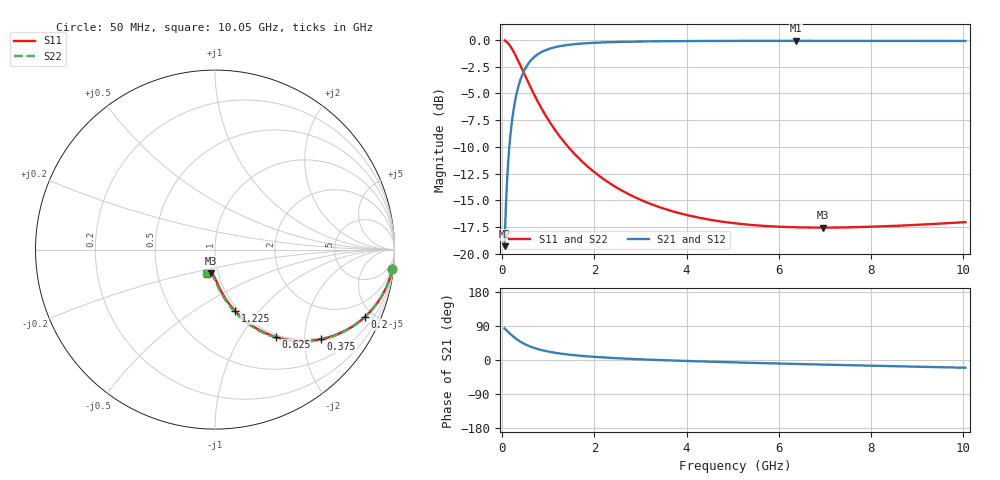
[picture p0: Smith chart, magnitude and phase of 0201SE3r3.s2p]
! AVX Thin Film Operation		Date: August 2001
! Description: Accu-P® Series, Thin Film, SMD, RF Capacitor
! Part Number: 0201YJ3R3ABW
! 50 MHz  -  10.05 GHz
! Serial Measurements
# mhz S db R 50
!	S11		S21		S12		S22
!	dB	Phase	dB	Phase	dB	Phase	dB	Phase
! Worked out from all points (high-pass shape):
!   401 points, 50 MHz to 10.05 GHz, reference 50 ohm
!   highest |S21| = -0.09 dB at 6.375 GHz (marker M1); lowest = -19.3 dB at 50 MHz (marker M2)
!   |S21| within 3 dB of the highest: 451.6 MHz to end of sweep
!   lowest |S11| = -17.5 dB at 6.95 GHz (marker M3), VSWR 1.31, Z = 46.1 - j12.2 ohm
!   |S11| at or under -10 dB: 1.431 GHz to end of sweep
!   |S22| runs from -17.5 to -0.1 dB; largest |S21 - S12| = 0
!   S11 on the Smith chart (normalised r, x): 50 MHz: 1, -18; 200 MHz: 0.96, -4.48; 375 MHz: 0.96, -2.40; 625 MHz: 0.96, -1.44; 1.225 GHz: 0.96, -0.75; 10.05 GHz: 0.88, -0.24
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50  -0.05 -6.4  -19.27 83.6  -19.27 83.6  -0.05 -6.4
100  -0.20 -12.6  -13.40 77.4  -13.40 77.4  -0.20 -12.7
125  -0.32 -15.6  -11.58 74.3  -11.58 74.3  -0.32 -15.7
150  -0.45 -18.5  -10.13 71.4  -10.13 71.4  -0.45 -18.6
200  -0.76 -24.1  -7.95 65.8  -7.95 65.8  -0.76 -24.2
275  -1.34 -31.7  -5.77 58.2  -5.77 58.2  -1.34 -31.9
375  -2.23 -40.2  -3.97 49.6  -3.97 49.6  -2.23 -40.5
500  -3.40 -48.7  -2.66 41.1  -2.66 41.1  -3.40 -49.0
625  -4.54 -55.2  -1.89 34.6  -1.89 34.6  -4.54 -55.6
750  -5.60 -60.2  -1.41 29.5  -1.41 29.5  -5.60 -60.7
875  -6.58 -64.2  -1.08 25.5  -1.08 25.5  -6.58 -64.8
1225  -8.89 -72.0  -0.61 17.6  -0.61 17.6  -8.89 -72.7
1725  -11.33 -78.5  -0.34 10.8  -0.34 10.8  -11.33 -79.6
2500  -13.84 -84.5  -0.19 4.6  -0.19 4.6  -13.84 -85.9
3400  -15.61 -89.0  -0.13 -0.1  -0.13 -0.1  -15.61 -90.8
4175  -16.53 -92.1  -0.10 -3.3  -0.10 -3.3  -16.53 -94.0
5050  -17.14 -95.0  -0.09 -6.4  -0.09 -6.4  -17.14 -97.0
6375  -17.51 -99.0  -0.09 -10.5  -0.09 -10.5  -17.51 -101.1
6725  -17.53 -100.0  -0.09 -11.5  -0.09 -11.5  -17.53 -102.1
6950  -17.54 -100.6  -0.09 -12.1  -0.09 -12.1  -17.54 -102.7
8400  -17.39 -104.6  -0.09 -16.1  -0.09 -16.1  -17.39 -106.5
10050  -17.02 -108.9  -0.10 -20.4  -0.10 -20.4  -17.02 -110.8
